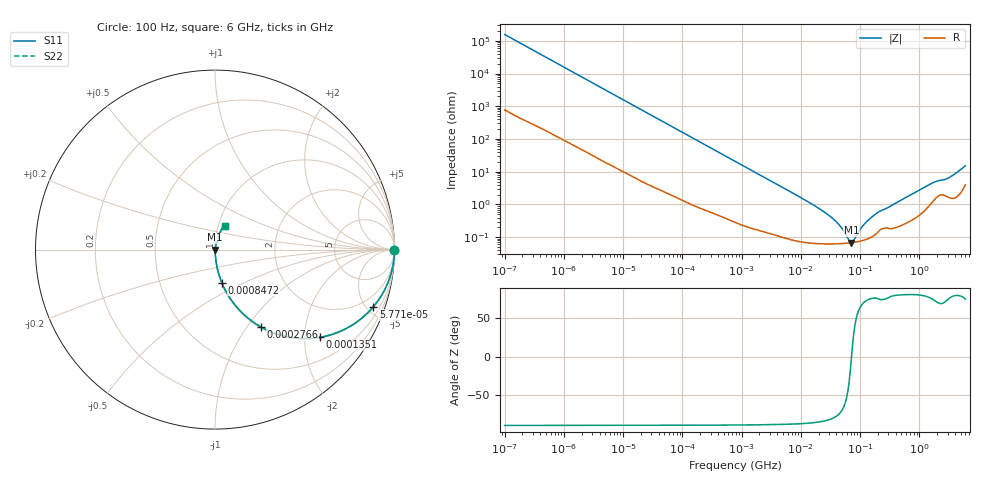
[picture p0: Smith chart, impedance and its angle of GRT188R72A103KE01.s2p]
!Murata Part Number: GRT188R72A103KE01
!These Parameters are Measured in Series Mode Connection
!Data Generated on Jun 19, 2026
!  o--ll--o
!Port1  Port2
!  o------o
!Operation Temp=25[degC], DC Bias Voltage=0[V]
!Freq. Start=100[Hz] Stop=6[GHz] 401[Steps]
# Hz S RI R 50
!Freq.(Hz) S11(Real) S11(Imag) S21(Real) S21(Imag) S12(Real) S12(Imag) S22(Real) S22(Imag)
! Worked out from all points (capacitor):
!   401 points, 100 Hz to 6 GHz, reference 50 ohm
!   read as one part in series: C = 10.2 nF near 109 Hz
!   lowest |Z| = 68 mohm at 71.29 MHz (marker M1)
!   series resonance near 71.8 MHz, so ESL is about 480 pH
!   S11 on the Smith chart (normalised r, x): 100 Hz: open; 57.71 kHz: 1.04, -5.53; 135.1 kHz: 1.02, -2.37; 276.6 kHz: 1.01, -1.16; 847.2 kHz: 1.01, -0.38; 6 GHz: 1.08, +0.29
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100  1 -0.000642  3.6e-06 0.000642  3.6e-06 0.000642  1 -0.000642
2008  0.9998 -0.0128  0.00024 0.0128  0.00024 0.0128  0.9998 -0.0128
12041  0.9938 -0.0754  0.00621 0.0754  0.00621 0.0754  0.9938 -0.0754
40335  0.9382 -0.2371  0.0618 0.2371  0.0618 0.2371  0.9382 -0.2371
57709  0.8824 -0.3183  0.1176 0.3183  0.1176 0.3183  0.8824 -0.3183
135116  0.5837 -0.4886  0.4163 0.4886  0.4163 0.4886  0.5837 -0.4886
276587  0.2549 -0.4306  0.7451 0.4306  0.7451 0.4306  0.2549 -0.4306
774597  0.0444 -0.1993  0.9556 0.1993  0.9556 0.1993  0.0444 -0.1993
847162  0.0377 -0.1836  0.9623 0.1836  0.9623 0.1836  0.0377 -0.1836
2713602  0.00496 -0.0598  0.995 0.0598  0.995 0.0598  0.00496 -0.0598
1.555665e7  0.000756 -0.0101  0.9992 0.0101  0.9992 0.0101  0.000756 -0.0101
3.80911e7  0.000637 -0.00312  0.9994 0.00312  0.9994 0.00312  0.000637 -0.00312
6.518806e7  0.000666 -0.000445  0.9993 0.000445  0.9993 0.000445  0.000666 -0.000445
7.129496e7  0.000679 -3.21e-05  0.9993 3.21e-05  0.9993 3.21e-05  0.000679 -3.21e-05
7.797396e7  0.000694 0.000381  0.9993 -0.000381  0.9993 -0.000381  0.000694 0.000381
1.066761e8  0.000782 0.00187  0.9992 -0.00187  0.9992 -0.00187  0.000782 0.00187
1.395531e8  0.000924 0.00329  0.9991 -0.00329  0.9991 -0.00329  0.000924 0.00329
1.996653e8  0.00146 0.00552  0.9985 -0.00552  0.9985 -0.00552  0.00146 0.00552
3.124326e8  0.0019 0.00822  0.9981 -0.00822  0.9981 -0.00822  0.0019 0.00822
1.565993e9  0.012 0.0408  0.988 -0.0408  0.988 -0.0408  0.012 0.0408
3.065283e9  0.0199 0.0591  0.9801 -0.0591  0.9801 -0.0591  0.0199 0.0591
6e9  0.0572 0.1333  0.9428 -0.1333  0.9428 -0.1333  0.0572 0.1333
